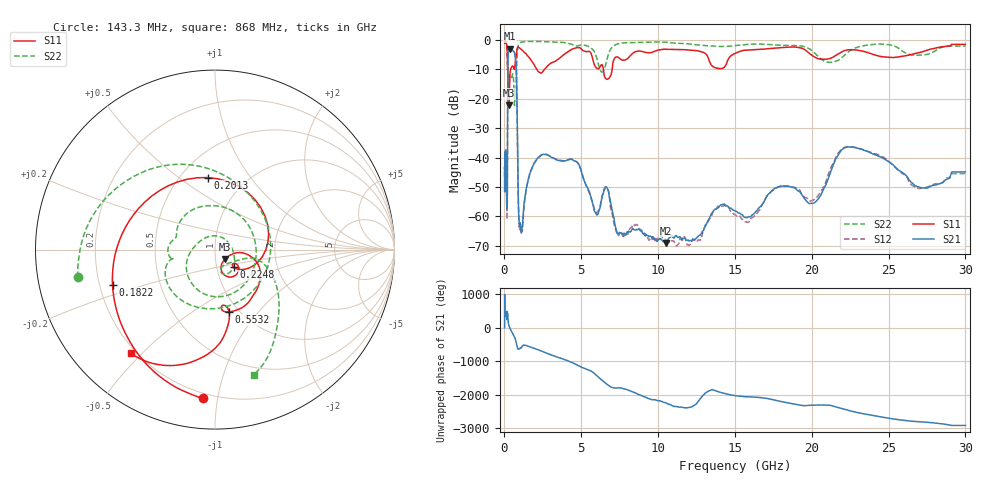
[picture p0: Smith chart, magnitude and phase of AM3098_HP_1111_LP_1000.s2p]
! Date/Time: Thu, Feb 28, 2019 8:47 AM
! Network Analyzer: Agilent Technologies E8364B Rev: A.07.50.67
! Sweep from 0.010 to 30.000 GHz, 1601 Points, Sweep Type: LOG
! Power Supply: 5.022 V, 0.002 A
# Hz S DB R 50
!freq MagS11 AngS11 MagS21 AngS21 MagS12 AngS12 MagS22 AngS22
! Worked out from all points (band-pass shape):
!   1601 points, 10 MHz to 30 GHz, reference 50 ohm
!   highest |S21| = -3.02 dB at 340.5 MHz (marker M1); lowest = -69.0 dB at 10.49 GHz (marker M2)
!   |S21| within 3 dB of the highest: 228.4 MHz to 708.3 MHz (479.9 MHz wide, 102 % of centre)
!   lowest |S11| = -22.2 dB at 293 MHz (marker M3), VSWR 1.17, Z = 55.5 - j5.98 ohm
!   |S11| at or under -10 dB: 210.2 MHz to 405.2 MHz (195 MHz wide, 63.4 % of centre); 2.095 GHz to 2.618 GHz (522.8 MHz wide, 22.2 % of centre); 6.438 GHz to 7.009 GHz (571 MHz wide, 8.49 % of centre)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
!   |S22| runs from -22.3 to -0.5 dB; largest |S21 - S12| = 0.012
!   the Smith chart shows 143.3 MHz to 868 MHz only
!   S11 on the Smith chart (normalised r, x): 143.3 MHz: 0.17, -0.91; 182.2 MHz: 0.25, -0.16; 201.3 MHz: 0.67, +0.64; 224.8 MHz: 1.20, -0.24; 553.2 MHz: 0.90, -0.71; 868 MHz: 0.18, -0.46
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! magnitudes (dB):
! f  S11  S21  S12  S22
! 10 MHz  -0.4  -43.4  -46.9  -0.6
! 38.04 MHz  -0.3  -40.9  -40.8  -0.6
! 143.3 MHz  -1.6  -53.9  -53.7  -2.1
! 144.7 MHz  -1.6  -55.0  -55.0  -2.2
! 182.2 MHz  -4.4  -55.9  -57.8  -5.8
! 201.3 MHz  -7.9  -30.5  -30.2  -10.2
! 224.8 MHz  -16.9  -6.9  -6.9  -11.6
! 293 MHz  -22.2  -3.2  -3.2  -12.7
! 340.5 MHz  -13.1  -3.0  -3.0  -12.3
! 550.5 MHz  -9.0  -3.8  -3.7  -11.6
! 553.2 MHz  -9.0  -3.8  -3.7  -11.6
! 758.3 MHz  -5.4  -9.4  -9.3  -18.2
! 868 MHz  -2.6  -42.8  -43.0  -2.7
! 954.5 MHz  -2.6  -61.9  -62.8  -1.2
! 1.126 GHz  -3.4  -64.6  -64.7  -0.8
! 2.084 GHz  -9.9  -40.7  -40.8  -0.6
! 4.663 GHz  -2.8  -41.3  -41.3  -2.1
! 7.926 GHz  -6.7  -65.8  -66.2  -1.0
! 10.49 GHz  -3.2  -69.0  -69.4  -0.8
! 20.1 GHz  -5.6  -55.5  -54.5  -4.1
! 22.56 GHz  -3.4  -36.4  -36.3  -3.5
! 30 GHz  -1.6  -44.9  -45.5  -2.2
